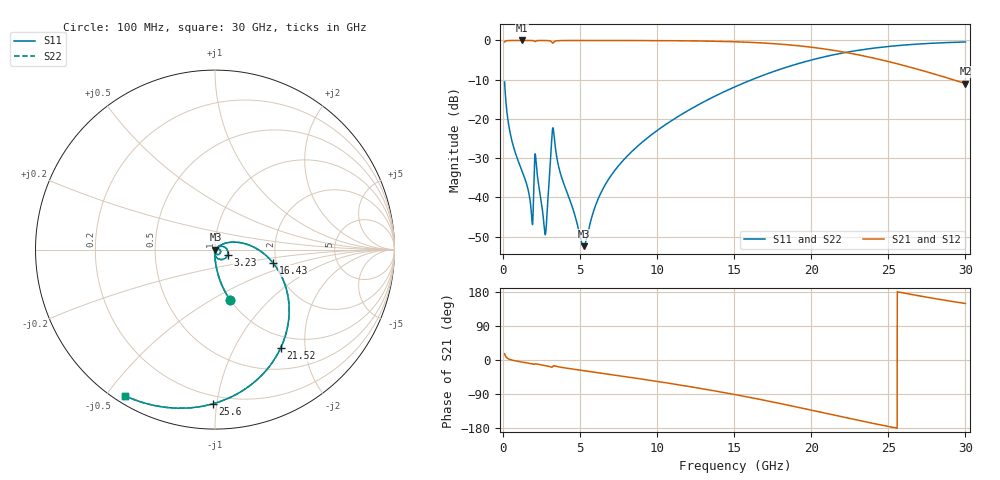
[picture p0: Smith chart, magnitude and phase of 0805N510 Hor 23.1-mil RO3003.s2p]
# GHz S MA R 50
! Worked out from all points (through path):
!   3201 points, 100 MHz to 30 GHz, reference 50 ohm
!   highest |S21| = -0.01 dB at 1.212 GHz (marker M1); lowest = -11.0 dB at 30 GHz (marker M2)
!   group delay of S21, straight-line fit = 20.4 ps
!   lowest |S11| = -52.4 dB at 5.22 GHz (marker M3), VSWR 1.00, Z = 50.2 - j0.115 ohm
!   |S11| at or under -10 dB: start of sweep to 16.15 GHz
!   |S22| runs from -52.4 to -0.4 dB; largest |S21 - S12| = 0
!   S11 on the Smith chart (normalised r, x): 100 MHz: 0.99, -0.62; 3.23 GHz: 1.15, -0.07; 16.43 GHz: 1.92, -0.32; 21.52 GHz: 0.80, -1.56; 25.6 GHz: 0.15, -0.98; 30 GHz: 0.03, -0.56
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0.1  0.2954 -73.3  0.9551 16.6  0.9551 16.6  0.2954 -73.3
0.511125  0.05931 -88.8  0.9976 0.6  0.9976 0.6  0.05931 -88.8
1.211906  0.02211 -92.9  0.9988 -5.3  0.9988 -5.3  0.02211 -92.9
1.828594  0.006652 -79.1  0.9976 -9.6  0.9976 -9.6  0.006652 -79.1
2.174313  0.02367 -77.7  0.9905 -10.5  0.9905 -10.5  0.02367 -77.7
2.725594  0.003377 -33.5  0.9967 -14.7  0.9967 -14.7  0.003377 -33.5
2.847062  0.005916 26.3  0.9955 -15.6  0.9955 -15.6  0.005916 26.3
3.108687  0.03783 29.2  0.974 -18.4  0.974 -18.4  0.03783 29.2
3.230156  0.07679 -23.6  0.9236 -17.0  0.9236 -17.0  0.07679 -23.6
3.725375  0.02005 -95.6  0.995 -19.0  0.995 -19.0  0.02005 -95.6
5.089563  0.002702 -54.9  0.9974 -27.3  0.9974 -27.3  0.002702 -54.9
5.220375  0.002386 -28.8  0.9974 -28.0  0.9974 -28.0  0.002386 -28.8
6.070656  0.008556 40.5  0.9973 -33.0  0.9973 -33.0  0.008556 40.5
6.874219  0.01733 43.9  0.9971 -37.7  0.9971 -37.7  0.01733 43.9
10.06978  0.07277 30.5  0.9938 -57.0  0.9938 -57.0  0.07277 30.5
15.05  0.2565 -2.4  0.9611 -91.3  0.9611 -91.3  0.2565 -2.4
16.43287  0.3326 -13.0  0.937 -102.1  0.937 -102.1  0.3326 -13.0
20.03956  0.565 -43.4  0.8174 -132.7  0.8174 -132.7  0.565 -43.4
21.51588  0.6598 -56.4  0.7431 -145.7  0.7431 -145.7  0.6598 -56.4
25.01978  0.8376 -86.1  0.5366 -175.6  0.5366 -175.6  0.8376 -86.1
25.59909  0.8588 -90.7  0.5025 179.8  0.5025 179.8  0.8588 -90.7
30  0.9558 -121.4  0.282 149.1  0.282 149.1  0.9558 -121.4
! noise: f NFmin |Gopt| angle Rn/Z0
0.1  0.0004097  0.8537  0.7659  0.0005977
3.417  0.01754  0.8822  18.49  0.03143
6.743  0.009896  0.6464  35.91  0.004824
10.06  0.0136  0.6297  52.29  0.00562
13.39  0.01788  0.6349  67.62  0.006506
16.7  0.02306  0.6537  81.84  0.007476
20.03  0.02975  0.6832  95.26  0.008618
23.35  0.03887  0.722  108.1  0.01003
26.67  0.05216  0.7687  120.7  0.01182
30  0.07292  0.8202  133.4  0.01398
